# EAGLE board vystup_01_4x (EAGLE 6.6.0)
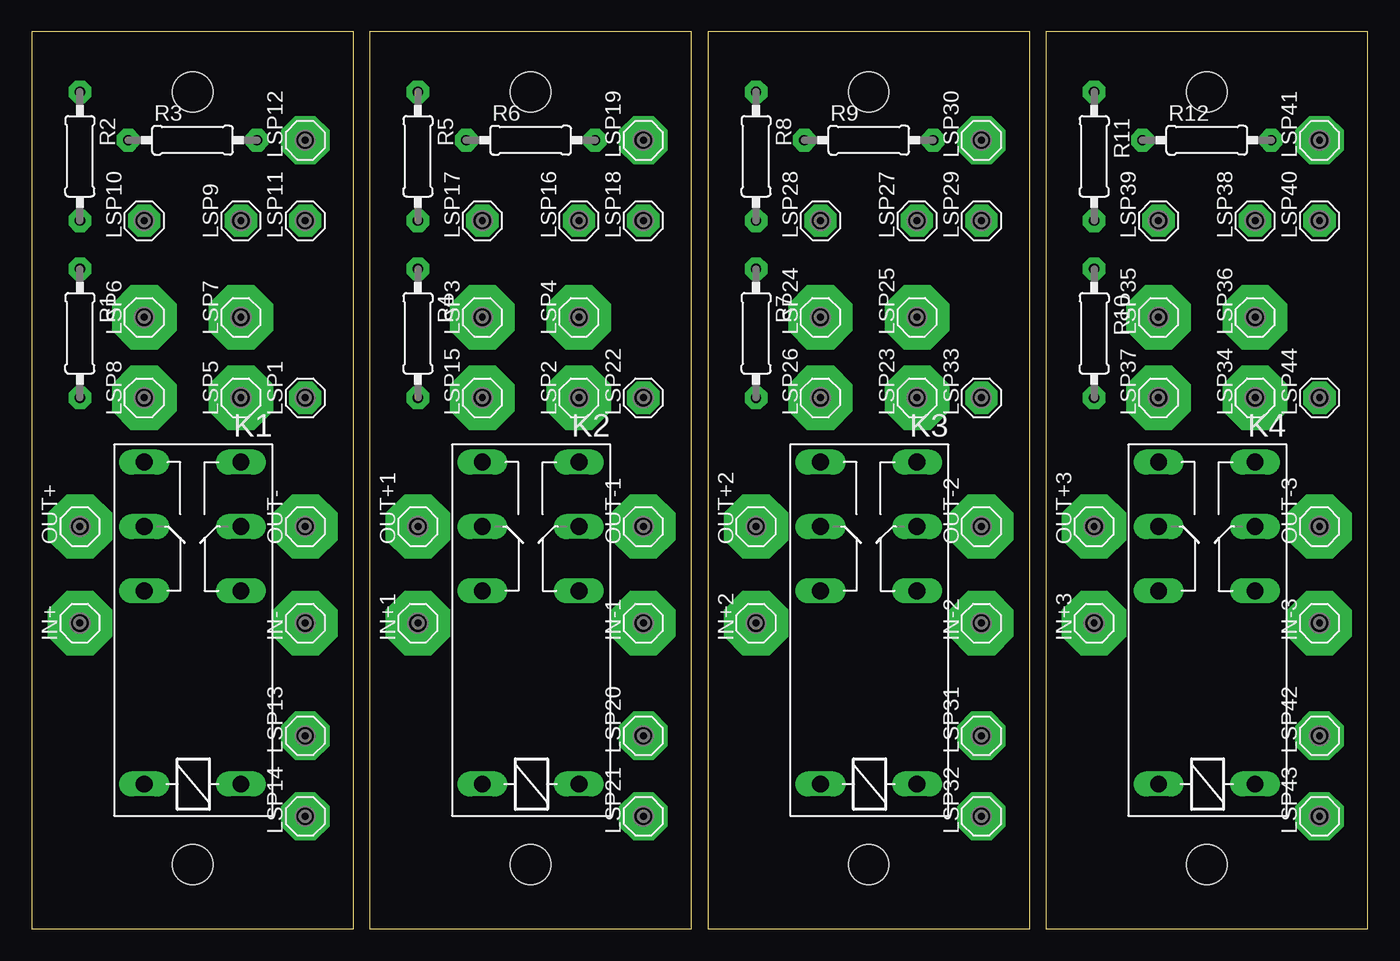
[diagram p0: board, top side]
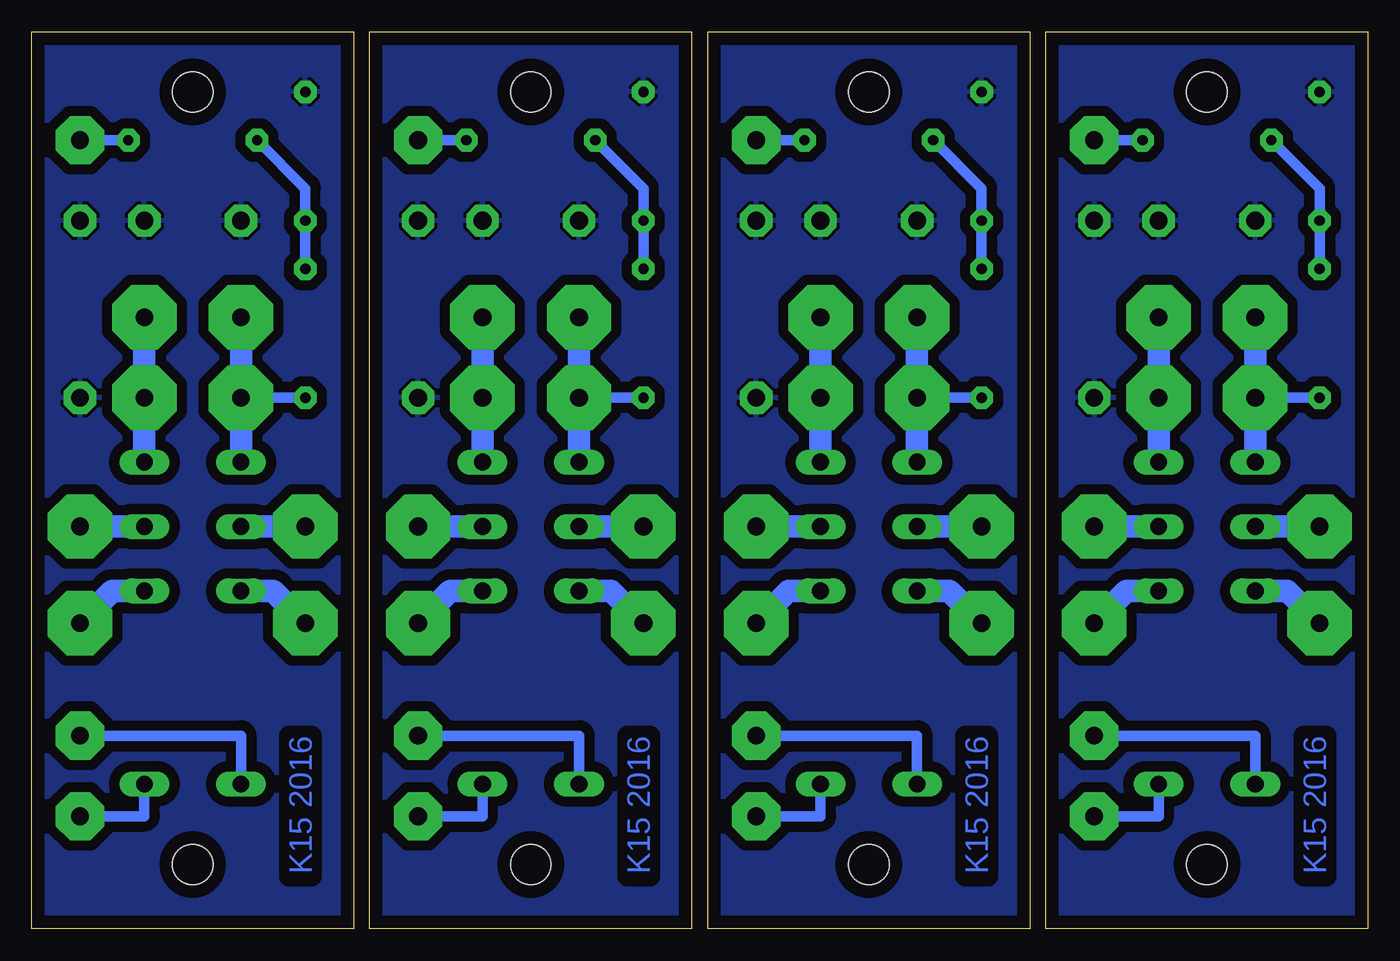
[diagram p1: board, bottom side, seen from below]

Size 105.4 x 70.79 mm. Coordinates in mm from the lower left corner, seen from the top.
Outline: 25.39,0 25.39,70.79 0,70.79 0,0 25.39,0
Outline: 52.06,0 52.06,70.79 26.67,70.79 26.67,0 52.06,0
Outline: 78.73,0 78.73,70.79 53.34,70.79 53.34,0 78.73,0
Outline: 105.4,0 105.4,70.79 80.01,70.79 80.01,0 105.4,0
Copper layers (1*16): Top 0.035mm / dielectric 1.5mm / Bottom 0.035mm
Design rules "default": minimum track width 10mil, minimum drill 24mil, track to track 8mil, track to pad 8mil, pad to pad 8mil, via to via 8mil, smd to smd 8mil, copper to edge 40mil, drill to drill 8mil, minimum pad ring 10mil, minimum via ring 8mil, stop-mask expansion 4mil, vias tented up to drill 0mil, thermal gap 10mil
Holes 3.2 mm at 12.69,5.08 12.69,66.04 39.36,5.08 39.36,66.04 66.03,5.08 66.03,66.04 92.7,5.08 92.7,66.04

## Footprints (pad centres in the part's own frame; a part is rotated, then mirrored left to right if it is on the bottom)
SE14 = drill 1.397 pad 2.54 octagon: MP 0,0
F4052 = drill 1.321 long: 1 -3.81,3.81; 2 -3.81,-3.81; O1 11.43,-3.81; O2 11.43,3.81; P1 16.51,-3.81; P2 16.51,3.81; S1 21.59,-3.81; S2 21.59,3.81
0207/10 = drill 0.813 pad 1.778 octagon: 1 -5.08,0; 2 5.08,0

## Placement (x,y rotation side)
IN+  SE14  [SE14]  3.8,24.13 90 top
IN+1  SE14  [SE14]  30.47,24.13 90 top
IN+2  SE14  [SE14]  57.14,24.13 90 top
IN+3  SE14  [SE14]  83.81,24.13 90 top
IN-  SE14  [SE14]  21.58,24.13 90 top
IN-1  SE14  [SE14]  48.25,24.13 90 top
IN-2  SE14  [SE14]  74.92,24.13 90 top
IN-3  SE14  [SE14]  101.59,24.13 90 top
K1  4052  [F4052]  12.69,15.24 90 top
K2  4052  [F4052]  39.36,15.24 90 top
K3  4052  [F4052]  66.03,15.24 90 top
K4  4052  [F4052]  92.7,15.24 90 top
LSP1  SE14  [SE14]  21.58,41.91 90 top
LSP2  SE14  [SE14]  43.17,41.91 90 top
LSP3  SE14  [SE14]  35.55,48.26 90 top
LSP4  SE14  [SE14]  43.17,48.26 90 top
LSP5  SE14  [SE14]  16.5,41.91 90 top
LSP6  SE14  [SE14]  8.88,48.26 90 top
LSP7  SE14  [SE14]  16.5,48.26 90 top
LSP8  SE14  [SE14]  8.88,41.91 90 top
LSP9  SE14  [SE14]  16.5,55.88 90 top
LSP10  SE14  [SE14]  8.88,55.88 90 top
LSP11  SE14  [SE14]  21.58,55.88 90 top
LSP12  SE14  [SE14]  21.58,62.23 90 top
LSP13  SE14  [SE14]  21.58,15.24 90 top
LSP14  SE14  [SE14]  21.58,8.89 90 top
LSP15  SE14  [SE14]  35.55,41.91 90 top
LSP16  SE14  [SE14]  43.17,55.88 90 top
LSP17  SE14  [SE14]  35.55,55.88 90 top
LSP18  SE14  [SE14]  48.25,55.88 90 top
LSP19  SE14  [SE14]  48.25,62.23 90 top
LSP20  SE14  [SE14]  48.25,15.24 90 top
LSP21  SE14  [SE14]  48.25,8.89 90 top
LSP22  SE14  [SE14]  48.25,41.91 90 top
LSP23  SE14  [SE14]  69.84,41.91 90 top
LSP24  SE14  [SE14]  62.22,48.26 90 top
LSP25  SE14  [SE14]  69.84,48.26 90 top
LSP26  SE14  [SE14]  62.22,41.91 90 top
LSP27  SE14  [SE14]  69.84,55.88 90 top
LSP28  SE14  [SE14]  62.22,55.88 90 top
LSP29  SE14  [SE14]  74.92,55.88 90 top
LSP30  SE14  [SE14]  74.92,62.23 90 top
LSP31  SE14  [SE14]  74.92,15.24 90 top
LSP32  SE14  [SE14]  74.92,8.89 90 top
LSP33  SE14  [SE14]  74.92,41.91 90 top
LSP34  SE14  [SE14]  96.51,41.91 90 top
LSP35  SE14  [SE14]  88.89,48.26 90 top
LSP36  SE14  [SE14]  96.51,48.26 90 top
LSP37  SE14  [SE14]  88.89,41.91 90 top
LSP38  SE14  [SE14]  96.51,55.88 90 top
LSP39  SE14  [SE14]  88.89,55.88 90 top
LSP40  SE14  [SE14]  101.59,55.88 90 top
LSP41  SE14  [SE14]  101.59,62.23 90 top
LSP42  SE14  [SE14]  101.59,15.24 90 top
LSP43  SE14  [SE14]  101.59,8.89 90 top
LSP44  SE14  [SE14]  101.59,41.91 90 top
OUT+  SE14  [SE14]  3.8,31.75 90 top
OUT+1  SE14  [SE14]  30.47,31.75 90 top
OUT+2  SE14  [SE14]  57.14,31.75 90 top
OUT+3  SE14  [SE14]  83.81,31.75 90 top
OUT-  SE14  [SE14]  21.58,31.75 90 top
OUT-1  SE14  [SE14]  48.25,31.75 90 top
OUT-2  SE14  [SE14]  74.92,31.75 90 top
OUT-3  SE14  [SE14]  101.59,31.75 90 top
R1  100  [0207/10]  3.8,46.99 270 top
R2  120  [0207/10]  3.8,60.96 270 top
R3  47  [0207/10]  12.69,62.23 0 top
R4  100  [0207/10]  30.47,46.99 270 top
R5  120  [0207/10]  30.47,60.96 270 top
R6  47  [0207/10]  39.36,62.23 0 top
R7  100  [0207/10]  57.14,46.99 270 top
R8  120  [0207/10]  57.14,60.96 270 top
R9  47  [0207/10]  66.03,62.23 0 top
R10  100  [0207/10]  83.81,46.99 270 top
R11  120  [0207/10]  83.81,60.96 270 top
R12  47  [0207/10]  92.7,62.23 0 top

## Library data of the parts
IN+ IN+1-IN+3 IN- IN-1-IN-3 LSP1-LSP44 OUT+ OUT+1-OUT+3 OUT- OUT-1-OUT-3 = solpad
K1-K4 = relay; OC_FARNELL: unknown; OC_NEWARK: unknown
R1-R12 = rcl

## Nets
GND: LSP1.MP LSP9.MP LSP10.MP LSP11.MP R2.1
GND1: LSP16.MP LSP17.MP LSP18.MP LSP22.MP R5.1
GND2: LSP27.MP LSP28.MP LSP29.MP LSP33.MP R8.1
GND3: LSP38.MP LSP39.MP LSP40.MP LSP44.MP R11.1
N$1: K1.S1 LSP5.MP LSP7.MP
N$2: K1.S2 LSP6.MP LSP8.MP R1.2
N$4: K1.P1 OUT-.MP
N$5: K1.P2 OUT+.MP
N$6: IN-.MP K1.O1
N$7: IN+.MP K1.O2
N$8: R1.1 R2.2 R3.1
N$9: LSP12.MP R3.2
N$10: K1.1 LSP13.MP
N$11: K1.2 LSP14.MP
N$18: K2.S1 LSP2.MP LSP4.MP
N$19: K2.S2 LSP3.MP LSP15.MP R4.2
N$20: K2.P1 OUT-1.MP
N$21: K2.P2 OUT+1.MP
N$22: IN-1.MP K2.O1
N$23: IN+1.MP K2.O2
N$24: R4.1 R5.2 R6.1
N$25: LSP19.MP R6.2
N$26: K2.1 LSP20.MP
N$27: K2.2 LSP21.MP
N$35: K3.S1 LSP23.MP LSP25.MP
N$36: K3.S2 LSP24.MP LSP26.MP R7.2
N$37: K3.P1 OUT-2.MP
N$38: K3.P2 OUT+2.MP
N$39: IN-2.MP K3.O1
N$40: IN+2.MP K3.O2
N$41: R7.1 R8.2 R9.1
N$42: LSP30.MP R9.2
N$43: K3.1 LSP31.MP
N$44: K3.2 LSP32.MP
N$52: K4.S1 LSP34.MP LSP36.MP
N$53: K4.S2 LSP35.MP LSP37.MP R10.2
N$54: K4.P1 OUT-3.MP
N$55: K4.P2 OUT+3.MP
N$56: IN-3.MP K4.O1
N$57: IN+3.MP K4.O2
N$58: R10.1 R11.2 R12.1
N$59: LSP41.MP R12.2
N$60: K4.1 LSP42.MP
N$61: K4.2 LSP43.MP

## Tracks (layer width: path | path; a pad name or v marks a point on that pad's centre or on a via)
GND
  pour Bottom (isolate 0.813): -0.01,0 -0.01,71.12 25.39,71.12 25.39,0
GND1
  pour Bottom (isolate 0.813): 26.66,0 26.66,71.12 52.06,71.12 52.06,0
GND2
  pour Bottom (isolate 0.813): 53.33,0 53.33,71.12 78.73,71.12 78.73,0
GND3
  pour Bottom (isolate 0.813): 80,0 80,71.12 105.4,71.12 105.4,0
N$1  (via drill 0.6 pad 5.08)
  Bottom 1.778: K1.S1 LSP5.MP LSP7.MP
  other vias: 16.5,48.26 16.5,41.91
N$2  (via drill 0.6 pad 5.08)
  Bottom 0.813: R1.2 LSP8.MP
  Bottom 1.778: K1.S2 LSP8.MP LSP6.MP
  other vias: 8.88,48.26 8.88,41.91
N$3  (via drill 0.6 pad 5.08)
  other vias: 3.8,24.13
N$4
  Bottom 1.778: OUT-.MP K1.P1
N$5
  Bottom 1.778: K1.P2 OUT+.MP
N$6
  Bottom 1.778: K1.O1 19.04,26.67 IN-.MP
N$7
  Bottom 1.778: K1.O2 6.34,26.67 IN+.MP
N$8
  Bottom 0.813: R1.1 R2.2 3.8,58.42 R3.1
N$9
  Bottom 0.813: R3.2 LSP12.MP
N$10
  Bottom 0.813: LSP13.MP 8.88,15.24 K1.1
N$11
  Bottom 0.813: LSP14.MP 16.5,8.89 K1.2
N$12  (via drill 0.6 pad 5.08)
  other vias: 3.8,31.75
N$13  (via drill 0.6 pad 5.08)
  other vias: 21.58,24.13
N$14  (via drill 0.6 pad 5.08)
  other vias: 21.58,31.75
N$15  (via drill 0.6 pad 3.81)
  other vias: 21.58,15.24
N$16  (via drill 0.6 pad 3.81)
  other vias: 21.58,8.89
N$17  (via drill 0.6 pad 3.81)
  other vias: 21.58,62.23
N$18  (via drill 0.6 pad 5.08)
  Bottom 1.778: K2.S1 LSP2.MP LSP4.MP
  other vias: 43.17,48.26 43.17,41.91
N$19  (via drill 0.6 pad 5.08)
  Bottom 0.813: R4.2 LSP15.MP
  Bottom 1.778: K2.S2 LSP15.MP LSP3.MP
  other vias: 35.55,48.26 35.55,41.91
N$20
  Bottom 1.778: OUT-1.MP K2.P1
N$21
  Bottom 1.778: K2.P2 OUT+1.MP
N$22
  Bottom 1.778: K2.O1 45.71,26.67 IN-1.MP
N$23
  Bottom 1.778: K2.O2 33.01,26.67 IN+1.MP
N$24
  Bottom 0.813: R4.1 R5.2 30.47,58.42 R6.1
N$25
  Bottom 0.813: R6.2 LSP19.MP
N$26
  Bottom 0.813: LSP20.MP 35.55,15.24 K2.1
N$27
  Bottom 0.813: LSP21.MP 43.17,8.89 K2.2
N$28  (via drill 0.6 pad 5.08)
  other vias: 30.47,24.13
N$29  (via drill 0.6 pad 5.08)
  other vias: 30.47,31.75
N$30  (via drill 0.6 pad 5.08)
  other vias: 48.25,24.13
N$31  (via drill 0.6 pad 5.08)
  other vias: 48.25,31.75
N$32  (via drill 0.6 pad 3.81)
  other vias: 48.25,15.24
N$33  (via drill 0.6 pad 3.81)
  other vias: 48.25,8.89
N$34  (via drill 0.6 pad 3.81)
  other vias: 48.25,62.23
N$35  (via drill 0.6 pad 5.08)
  Bottom 1.778: K3.S1 LSP23.MP LSP25.MP
  other vias: 69.84,48.26 69.84,41.91
N$36  (via drill 0.6 pad 5.08)
  Bottom 0.813: R7.2 LSP26.MP
  Bottom 1.778: K3.S2 LSP26.MP LSP24.MP
  other vias: 62.22,48.26 62.22,41.91
N$37
  Bottom 1.778: OUT-2.MP K3.P1
N$38
  Bottom 1.778: K3.P2 OUT+2.MP
N$39
  Bottom 1.778: K3.O1 72.38,26.67 IN-2.MP
N$40
  Bottom 1.778: K3.O2 59.68,26.67 IN+2.MP
N$41
  Bottom 0.813: R7.1 R8.2 57.14,58.42 R9.1
N$42
  Bottom 0.813: R9.2 LSP30.MP
N$43
  Bottom 0.813: LSP31.MP 62.22,15.24 K3.1
N$44
  Bottom 0.813: LSP32.MP 69.84,8.89 K3.2
N$45  (via drill 0.6 pad 5.08)
  other vias: 57.14,24.13
N$46  (via drill 0.6 pad 5.08)
  other vias: 57.14,31.75
N$47  (via drill 0.6 pad 5.08)
  other vias: 74.92,24.13
N$48  (via drill 0.6 pad 5.08)
  other vias: 74.92,31.75
N$49  (via drill 0.6 pad 3.81)
  other vias: 74.92,15.24
N$50  (via drill 0.6 pad 3.81)
  other vias: 74.92,8.89
N$51  (via drill 0.6 pad 3.81)
  other vias: 74.92,62.23
N$52  (via drill 0.6 pad 5.08)
  Bottom 1.778: K4.S1 LSP34.MP LSP36.MP
  other vias: 96.51,48.26 96.51,41.91
N$53  (via drill 0.6 pad 5.08)
  Bottom 0.813: R10.2 LSP37.MP
  Bottom 1.778: K4.S2 LSP37.MP LSP35.MP
  other vias: 88.89,48.26 88.89,41.91
N$54
  Bottom 1.778: OUT-3.MP K4.P1
N$55
  Bottom 1.778: K4.P2 OUT+3.MP
N$56
  Bottom 1.778: K4.O1 99.05,26.67 IN-3.MP
N$57
  Bottom 1.778: K4.O2 86.35,26.67 IN+3.MP
N$58
  Bottom 0.813: R10.1 R11.2 83.81,58.42 R12.1
N$59
  Bottom 0.813: R12.2 LSP41.MP
N$60
  Bottom 0.813: LSP42.MP 88.89,15.24 K4.1
N$61
  Bottom 0.813: LSP43.MP 96.51,8.89 K4.2
N$62  (via drill 0.6 pad 5.08)
  other vias: 83.81,24.13
N$63  (via drill 0.6 pad 5.08)
  other vias: 83.81,31.75
N$64  (via drill 0.6 pad 5.08)
  other vias: 101.59,24.13
N$65  (via drill 0.6 pad 5.08)
  other vias: 101.59,31.75
N$66  (via drill 0.6 pad 3.81)
  other vias: 101.59,15.24
N$67  (via drill 0.6 pad 3.81)
  other vias: 101.59,8.89
N$68  (via drill 0.6 pad 3.81)
  other vias: 101.59,62.23

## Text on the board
Bottom: K15 2016 | K15 2016 | K15 2016 | K15 2016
